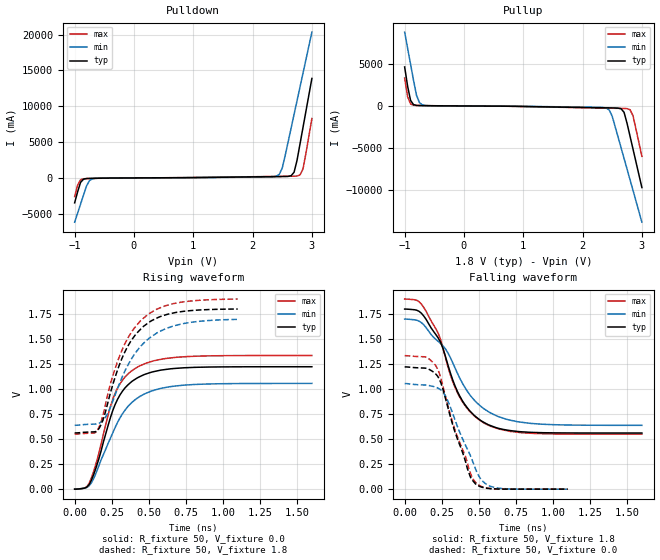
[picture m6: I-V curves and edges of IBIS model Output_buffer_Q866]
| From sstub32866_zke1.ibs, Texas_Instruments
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|   Model   Output_buffer_Q866
[Model]   Output_buffer_Q866
Model_type   Output
Polarity   Non-Inverting
Vmeas  =   0.90
Cref   =   30.0p
Rref   =   500
Vref   =   0.90
|Variable   typ   min   max
C_comp   1.922e-12   1.617e-12   2.952e-12
|Variable   typ   min   max
[Voltage range]   1.8   1.7   1.9
|Variable   typ   min   max
[Temperature range]  27   125   0.0
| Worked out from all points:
|   slope of the pulldown table from 0 to 0.27 V, typ, clamps not added: 22.5 ohm
|   slope of the pullup table from 0 to 0.27 V, typ, clamps not added: 23.6 ohm
|   rising waveform, R_fixture 50, V_fixture 0.0: 20-80 % time 171ps typ, 214ps min, 167ps max; typ from 0 V to 1.22 V
|   falling waveform, R_fixture 50, V_fixture 1.8: 20-80 % time 218ps typ, 279ps min, 216ps max; typ from 1.8 V to 0.561 V
|   rising waveform, R_fixture 50, V_fixture 1.8: 20-80 % time 201ps typ, 235ps min, 210ps max; typ from 0.561 V to 1.8 V
|   falling waveform, R_fixture 50, V_fixture 0.0: 20-80 % time 154ps typ, 174ps min, 170ps max; typ from 1.22 V to 0 V
[Pulldown]
|Voltage   I(typ)   I(min)   I(max)
-1V       -3.478A    -6.18A     -2.607A
-950mV    -1.947A    -4.915A    -1.011A
-900mV    -621.2mA   -3.652A    -262.6mA
-800mV    -88.75mA   -1.133A    -93.75mA
-700mV    -59.28mA   -123.8mA   -72.51mA
2.45V     188.7mA    499.5mA    214.5mA
2.5V      193.2mA    1.364A     219.5mA
2.65V     306.4mA    6.966A     234.3mA
2.7V      799.3mA    8.88A      241.1mA
2.8V      4.76A      12.71A     413.6mA
2.85V     7.044A     14.62A     1.259A
3V        13.9A      20.36A     8.287A
[Pullup]
|Voltage   I(typ)   I(min)   I(max)
-1V       4.646A     8.795A     3.323A
-950mV    2.359A     6.88A      1.107A
-900mV    662.3mA    4.966A     239.8mA
-800mV    64.07mA    1.269A     59.48mA
-750mV    46.28mA    394.4mA    51.82mA
-700mV    39.98mA    120.6mA    46.34mA
2.45V     -230mA     -489.1mA   -266.6mA
2.5V      -235.3mA   -1.234A    -272.5mA
2.7V      -764.8mA   -6.26A     -297.4mA
2.8V      -3.596A    -8.784A    -449.9mA
2.85V     -5.125A    -10.05A    -1.165A
3V        -9.723A    -13.84A    -5.997A
[Ramp]
|Variable   typ   min   max
dV/dt_r  0.7332/1.711e-10   0.6334/2.140e-10   0.8005/1.661e-10
dV/dt_f  0.7433/2.173e-10   0.6373/2.785e-10   0.8102/2.156e-10
R_load  =  50
[Rising Waveform]
R_fixture   =   50
V_fixture   =   0.0
V_fixture_min   =   0.0
V_fixture_max   =   0.0
C_fixture   =   0.00
|Time   V(typ)   V(min)   V(max)
0s        705nV      5.666uV    0V
96.97ps   44.49mV    32.27mV    57.13mV
145.5ps   219.1mV    164.4mV    261.3mV
226.3ps   638.7mV    457.9mV    745.8mV
274.7ps   851.1mV    620.6mV    962.9mV
339.4ps   1.01V      787.9mV    1.119V
420.2ps   1.109V     905.7mV    1.215V
533.3ps   1.173V     986.4mV    1.281V
727.3ps   1.211V     1.037V     1.32V
1.6ns     1.222V     1.056V     1.334V
[Falling Waveform]
R_fixture   =   50
V_fixture   =   1.8
V_fixture_min   =   1.7
V_fixture_max   =   1.9
C_fixture   =   0.00
|Time   V(typ)   V(min)   V(max)
0s        1.8V       1.7V       1.9V
80.81ps   1.789V     1.689V     1.888V
129.3ps   1.73V      1.642V     1.816V
242.4ps   1.466V     1.456V     1.495V
307.1ps   1.168V     1.319V     1.148V
371.7ps   930.3mV    1.11V      919.1mV
436.4ps   787.3mV    949.3mV    782mV
533.3ps   668.6mV    804.9mV    662.6mV
840.4ps   568.8mV    658.8mV    559.5mV
1.6ns     561.1mV    637.9mV    549.8mV
[Rising Waveform]
R_fixture   =   50
V_fixture   =   1.8
V_fixture_min   =   1.7
V_fixture_max   =   1.9
C_fixture   =   0.00
|Time   V(typ)   V(min)   V(max)
0s        561.1mV    637.8mV    549.7mV
155.6ps   588mV      651.8mV    592mV
188.9ps   682.4mV    685mV      725.8mV
222.2ps   853.3mV    754.6mV    940.4mV
266.7ps   1.088V     916.2mV    1.175V
322.2ps   1.316V     1.125V     1.397V
411.1ps   1.544V     1.362V     1.623V
500ps     1.663V     1.504V     1.751V
722.2ps   1.772V     1.65V      1.867V
1.1ns     1.798V     1.695V     1.898V
[Falling Waveform]
R_fixture   =   50
V_fixture   =   0.0
V_fixture_min   =   0.0
V_fixture_max   =   0.0
C_fixture   =   0.00
|Time   V(typ)   V(min)   V(max)
0s        1.222V     1.056V     1.334V
144.4ps   1.209V     1.04V      1.319V
222.2ps   1.13V      1.012V     1.202V
277.8ps   894.2mV    924.8mV    912mV
333.3ps   599.8mV    718.3mV    619.8mV
433.3ps   163mV      368.6mV    206.1mV
488.9ps   41.63mV    163.3mV    53.01mV
544.4ps   11.75mV    56.36mV    14.45mV
611.1ps   2.467mV    15.22mV    3.019mV
1.1ns     0V         0V         0V
